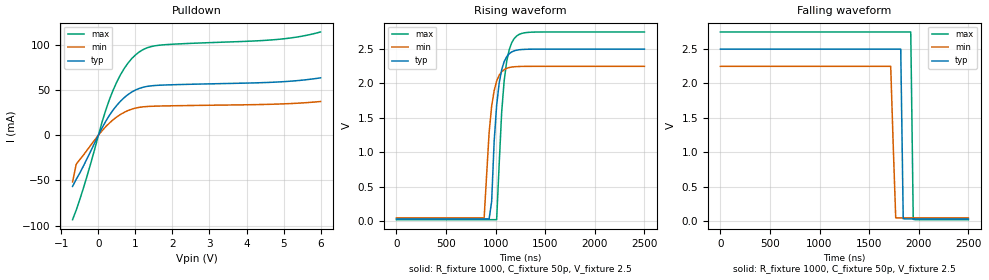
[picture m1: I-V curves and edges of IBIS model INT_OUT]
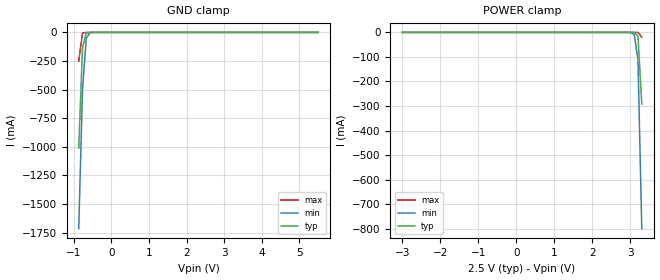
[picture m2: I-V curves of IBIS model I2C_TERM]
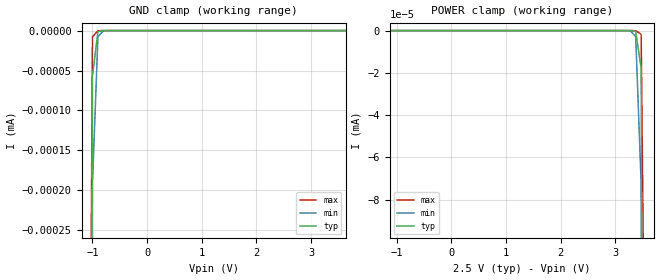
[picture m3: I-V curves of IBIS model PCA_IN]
|   NXP Semiconductors Inc.
|   Specialty Logic Products Group
|   IBIS model of PCA9545A
|   4-Channel I2C switch with
|   interrupt logic and reset
[IBIS Ver]   3.2
[Comment Char]   |_char
|  VDD Typ: 2.5V, Min: 2.25V, Max: 2.75V
[File name]   pca9545a_2_5v.ibs
[File Rev]   1.0
[Date]   Dec 05, 2007 9:30:50 AM
[Source]
Generated by Seshadri Venkataramanan with IbisToolKit at Tempe, AZ
[Notes]
[Disclaimer]
(C) Copyright 2007 NXP Semiconductors
All rights reserved
NXP Semiconductors (NXP) does not warrant that this model and any other
accompanying information (Model) accurately or fully represents the
operating characteristics and specifications of the semiconductor
products to which the Model relates.  Moreover, the Model is furnished
on an "as is" and with "all faults" basis, and without support or
warranty of any kind.  NXP disclaims all warranties, whether expressed
or implied or statutory, including without limitation all implied
warranties of non-infringement, merchantability and fitness for any
purpose, and those arising from a course of dealing or usage of trade.
NXP does not convey any license under its or any third party's patents,
copyrights or other intellectual property or proprietary rights.
You and your company assume any and all risks and liability arising out
of the application or use of the Model.
In no event shall NXP be liable for any direct, indirect, special,
consequential or incidental damages, however caused, whether in
warranty, contract or tort (including negligence), strict liability or
other legal theory, including, without limitation, for lost profits,
business interruption, or corruption or loss of data or information,
arising out of or in connection with the use of or the inability to use
the Model, even if NXP has been advised of the possibility of such
damages.
NXP provides the Model as a courtesy to our customers. You and your
company shall not distribute, convey, sell, or give the Model to anyone
else without receiving prior written permission from NXP.
NXP reserves the right to make changes without notice to the Model to
improve reliability, function, or design.
Please be aware that your receipt and subsequent use of the Model shall
serve as acceptance of these terms and conditions.  If you do not
accept these terms, return or destroy the Model immediately.
[Copyright]
2007
[Component]   PCA9545AD
Si_location Pin
Timing_location Pin
[Manufacturer]   NXP Semiconductors
[Package]
|   variable   typ   min   max
R_pkg   5.95E-02   5.36E-02   6.59E-02
L_pkg   4.21E-09   3.07E-09   5.91E-09
C_pkg   0.910E-12   0.758E-12   1.110E-12
|   SO20
[Pin] signal_name   model_name   R_pin   L_pin   C_pin
1   A0   PCA_IN   5.75E-02  5.91E-09  1.050E-12
2   A1   PCA_IN   6.25E-02  4.85E-09  1.040E-12
3   RESETB   PCA_IN   6.59E-02  3.92E-09  0.861E-12
4   INT0B   INT_IN   5.79E-02  3.32E-09  0.803E-12
5   SD0   I2C_TERM   5.36E-02  3.07E-09  0.758E-12
6   SC0   I2C_TERM   5.36E-02  3.07E-09  0.758E-12
7   INT1B   INT_IN   5.79E-02  3.32E-09  0.803E-12
8   SD1   I2C_TERM   6.59E-02  3.92E-09  0.861E-12
9   SC1   I2C_TERM   6.25E-02  4.85E-09  1.040E-12
10   Vss   GND   5.75E-02  5.91E-09  1.110E-12
11   INT2B   INT_IN   5.75E-02  5.91E-09  1.110E-12
12   SD2   I2C_TERM   6.25E-02  4.85E-09  1.040E-12
13   SC2   I2C_TERM   6.59E-02  3.92E-09  0.861E-12
14   INT3B   INT_IN   5.79E-02  3.32E-09  0.803E-12
15   SD3   I2C_TERM   5.36E-02  3.07E-09  0.758E-12
16   SC3   I2C_TERM   5.36E-02  3.07E-09  0.758E-12
17   INTB   INT_OUT   5.79E-02  3.32E-09  0.803E-12
18   SCL   I2C_TERM   6.59E-02  3.92E-09  0.861E-12
19   SDA   I2C_TERM   6.25E-02  4.85E-09  1.040E-12
20   Vdd   POWER   5.75E-02  5.91E-09  1.110E-12
[Component]   PCA9545APW
Si_location Pin
Timing_location Pin
[Manufacturer]   NXP Semiconductors
[Package]
|   variable   typ   min   max
R_pkg   7.24E-02   6.63E-02   8.34E-02
L_pkg   2.47E-09   2.09E-09   3.18E-09
C_pkg   0.341E-12   0.282E-12   0.420E-12
|   TSSOP20
[Pin] signal_name   model_name   R_pin   L_pin   C_pin
1   A0   PCA_IN   6.63E-02  3.18E-09  0.408E-12
2   A1   PCA_IN   6.67E-02  2.55E-09  0.398E-12
3   RESETB   PCA_IN   8.34E-02  2.35E-09  0.317E-12
4   INT0B   INT_IN   7.44E-02  2.16E-09  0.293E-12
5   SD0   I2C_TERM   7.10E-02  2.09E-09  0.282E-12
6   SC0   I2C_TERM   7.10E-02  2.09E-09  0.282E-12
7   INT1B   INT_IN   7.44E-02  2.16E-09  0.293E-12
8   SD1   I2C_TERM   8.34E-02  2.35E-09  0.317E-12
9   SC1   I2C_TERM   6.67E-02  2.55E-09  0.397E-12
10   Vss   GND   6.63E-02  3.18E-09  0.420E-12
11   INT2B   INT_IN   6.63E-02  3.17E-09  0.420E-12
12   SD2   I2C_TERM   6.67E-02  2.55E-09  0.397E-12
13   SC2   I2C_TERM   8.34E-02  2.35E-09  0.317E-12
14   INT3B   INT_IN   7.44E-02  2.16E-09  0.293E-12
15   SD3   I2C_TERM   7.10E-02  2.09E-09  0.282E-12
16   SC3   I2C_TERM   7.10E-02  2.09E-09  0.282E-12
17   INTB   INT_OUT   7.44E-02  2.16E-09  0.293E-12
18   SCL   I2C_TERM   8.34E-02  2.35E-09  0.317E-12
19   SDA   I2C_TERM   6.67E-02  2.55E-09  0.398E-12
20   Vdd   POWER   6.63E-02  3.17E-09  0.420E-12
[Component]   PCA9545ABS
Si_location Pin
Timing_location Pin
[Manufacturer]   NXP Semiconductors
[Package]
|   variable   typ   min   max
R_pkg   0.364   0.215   0.513
L_pkg   1.49E-09   1.04E-09   1.93E-09
C_pkg   0.149E-12   0.124E-12   0.173E-12
|   HVQFN20
[Package Model]   hvqfn20
[Pin] signal_name   model_name
1   RESETB   I2C_TERM
2   INT0B   INT_IN
3   SD0   I2C_TERM
4   SC0   I2C_TERM
5   INT1B   INT_IN
6   SD1   I2C_TERM
7   SC1   I2C_TERM
8   Vss   GND
9   INT2B   INT_IN
10   SD2   I2C_TERM
11   SC2   I2C_TERM
12   INT3B   INT_IN
13   SD3   I2C_TERM
14   SC3   I2C_TERM
15   INTB   INT_OUT
16   SCL   I2C_TERM
17   SDA   I2C_TERM
18   Vdd   POWER
19   A0   PCA_IN
20   A1   PCA_IN
[Series Pin Mapping] pin_2 model_name   function_table_group
18   6   PCA_SW   1
18   9   PCA_SW   2
18   13   PCA_SW   3
18   16   PCA_SW   4
19   5   PCA_SW   1
19   8   PCA_SW   2
19   12   PCA_SW   3
19   15   PCA_SW   4
[Series Switch Groups]
|   Function Group States
|  default
Off 1 2 3 4 /
On 1 /
On 2 /
On 3 /
On 4 /
[Define Package Model]   hvqfn20
[Manufacturer]   Unknown
[OEM]   Unknown
[Description]   none
[Number of Pins]   20
[Pin Numbers]
|   1 = RESETB
1
|   2 = INT0B
2
|   3 = SD0
3
|   4 = SC0
4
|   5 = INT1B
5
|   6 = SD1
6
|   7 = SC1
7
|   8 = VSS
8
|   9 = INT2B
9
|   10 = SD2
10
|   11 = SC2
11
|   12 = INT3B
12
|   13 = SD3
13
|   14 = SC3
14
|   15 = INTB
15
|   16 = SCL
16
|   17 = SDA
17
|   18 = VDD
18
|   19 = A0
19
|   20 = A1
20
[Model Data]
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[End Model Data]
[End Package Model]
[Model]   PCA_SW
Model_type Series_switch
C_comp   0.5p   0.5p   0.5p
[Temperature Range] 27   -40   85
[Voltage Range]   3.3   2.3   5.5
[Pullup Reference]  3.3   2.3   5.5
[Pulldown Reference]0   0   0
[On]
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[Off]
|   variable   R(typ)   R(min)   R(max)
[R Series]   1e06   1e06   1e06
|[End   PCA_SW
| [End   PCA_SW
| Models and submodels in the file (5): INT_OUT (Open_drain), I2C_TERM (Terminator), PCA_IN (Input), INT_IN (Input), PCA_SW (Series_switch)
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[Model]   INT_OUT
Model_type Open_drain
Vref=3.3
Vmeas=1.65
Rref=1000
Cref=1p
C_comp   2.2p   2p   2.3p
[Model Spec]
Vmeas   1.65   1.485   1.815
[Temperature Range] 27   85   -40
[Voltage Range]   2.5   2.25   2.75
[Pullup Reference]  2.5   2.25   2.75
[Pulldown Reference]0   0   0
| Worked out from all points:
|   slope of the pulldown table from 0 to 0.375 V, typ, clamps not added: 14.2 ohm
|   falling waveform, R_fixture 1000, C_fixture 50p, V_fixture 2.5: 20-80 % time 15.2ns typ, 30.3ns min, 15.2ns max; typ from 2.5 V to 0.029 V
|   rising waveform, R_fixture 1000, C_fixture 50p, V_fixture 2.5: 20-80 % time 68.9ns typ, 73.5ns min, 73.2ns max; typ from 0.029 V to 2.5 V
[Pulldown]
-700mV    -56.73mA   -51.78mA   -93.46mA
-600mV    -48.74mA   -32.17mA   -82.78mA
-300mV    -25.4mA    -16.24mA   -44.15mA
100mV     8.124mA    4.947mA    14.76mA
400mV     27.94mA    17.07mA    50.02mA
700mV     41.54mA    25.23mA    73.83mA
900mV     47.58mA    28.65mA    84.53mA
1.1V      51.52mA    30.64mA    91.81mA
1.3V      53.71mA    31.54mA    96.21mA
1.6V      54.98mA    32.05mA    99.08mA
4.7V      58.38mA    34.09mA    105.2mA
6V        63.25mA    37.12mA    113.9mA
[Falling Waveform]
R_fixture=1000
C_fixture=50p
V_fixture=2.5
V_fixture_min=2.25
V_fixture_max=2.75
0s        2.5V       2.25V      2.75V
1.717us   2.5V       2.25V      2.75V
1.742us   2.5V       1.106V     2.75V
1.768us   2.5V       44.5mV     2.75V
1.818us   2.5V       43.55mV    2.75V
1.843us   31.76mV    43.55mV    2.75V
1.919us   29.48mV    43.55mV    2.75V
1.944us   29.48mV    43.55mV    22.55mV
2.5us     29.47mV    43.55mV    17.78mV
[Rising Waveform]
R_fixture=1000
C_fixture=50p
V_fixture=2.5
V_fixture_min=2.25
V_fixture_max=2.75
0s        29.47mV    43.53mV    17.78mV
883.8ns   29.47mV    43.54mV    17.78mV
959.6ns   284mV      1.668V     17.79mV
984.8ns   1.155V     1.897V     17.79mV
1.01us    1.684V     2.036V     17.8mV
1.061us   2.2V       2.171V     1.581V
1.086us   2.318V     2.202V     2.042V
1.136us   2.433V     2.232V     2.49V
1.212us   2.485V     2.246V     2.692V
2.5us     2.5V       2.25V      2.75V
[Ramp]
R_load=1000
dV/dt_r   1.961E+0/1.306E-9   1.755E+0/1.384E-9   2.166E+0/1.192E-9
dV/dt_f   1.961E+0/7.920E-10   1.755E+0/1.468E-9   2.166E+0/6.141E-10
|[End   INT_OUT
| [End   I2C_TERM
|  [End   I2C_TERM
[Model]   I2C_TERM
Model_type Terminator
C_comp   9.5p   9.5p   9.5p
[Temperature Range] 27   85   -40
[Voltage Range]   2.5   2.25   2.75
[Pullup Reference]  2.5   2.25   2.75
[Pulldown Reference]0   0   0
[POWER Clamp Reference]2.5   2.25   2.75
[GND Clamp Reference]0   0   0
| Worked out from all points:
|   GND clamp passes 1 mA (typ) near -0.59 V on its own axis
[GND Clamp]
|   -6.000000E-1   -1.554225E-1   -1.242642E-1   -2.666059E-1
|   -5.000000E-1   -1.602113E-1   -1.179351E-1   -2.662641E-1
|   -4.000000E-1   -1.574088E-1   -1.099432E-1   -2.800035E-1
-870mV    -1.011A    -1.716A    -249.5mA
-770mV    -134.2mA   -501.1mA   -5.08mA
-670mV    -5.469mA   -51.14mA   -37.37uA
-570mV    -124.5uA   -3.038mA   -257.8nA
5.5V      803pA      906.4pA    802.9pA
[POWER Clamp]
-3V       803pA      906.4pA    802.9pA
2.9V      -174.5nA   -13.09uA   -133.3pA
3V        -8.329uA   -332.1uA   -8.003nA
3.1V      -395.1uA   -7.461mA   -1.147uA
3.2V      -15.49mA   -110.5mA   -166uA
3.3V      -291.7mA   -800mA     -19.51mA
[Model]   PCA_IN
Model_type Input
Vinh=2.1
Vinl=0.9
C_comp   1.73p   1.73p   1.73p
[Temperature Range] 27   85   -40
[Voltage Range]   2.5   2.25   2.75
[POWER Clamp Reference]2.5   2.25   2.75
[GND Clamp Reference]0   0   0
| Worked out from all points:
|   GND clamp passes 1 mA (typ) near -1.21 V on its own axis
[GND Clamp]
-3.3V     -35.52A    -34.27A    -37.05A
-1.1V     -2.718uA   -4.916uA   -1.14uA
-1V       -56.9nA    -192.5nA   -7.858nA
-900mV    -1.192nA   -7.538nA   -55.05pA
-800mV    -25.74pA   -295.9pA   -1.173pA
-700mV    -1.222pA   -12.26pA   -702.6fA
3.63V     3.63pA     3.63pA     3.63pA
[POWER Clamp]
-1.13V    3.63pA     3.63pA     3.63pA
3.17V     -833.7fA   -5.042pA   -670.6fA
3.27V     -8.589pA   -112.4pA   -853.8fA
3.37V     -374.3pA   -2.852nA   -13.03pA
3.47V     -17.84nA   -72.82nA   -1.766nA
3.57V     -852.2nA   -1.86uA    -256.1nA
5.77V     -34.93A    -33.68A    -36.46A
